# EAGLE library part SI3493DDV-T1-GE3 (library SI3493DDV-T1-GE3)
MOSFET -20V Vds 8V Vgs TSOP-6 Source: Datasheet
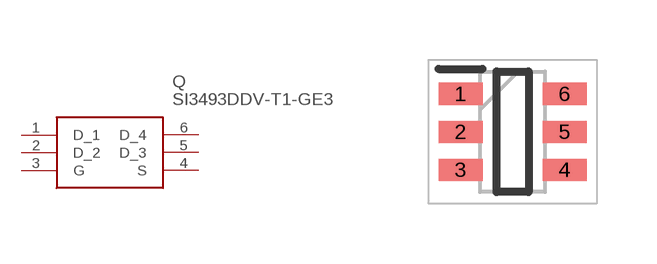
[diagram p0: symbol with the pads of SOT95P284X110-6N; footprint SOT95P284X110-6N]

Designator prefix Q

## SI3493DDV-T1-GE3 (Description: MOSFET -20V Vds 8V Vgs TSOP-6; Height: 1.1mm; Manufacturer_Name: Vishay; Manufacturer_Part_Number: SI3493DDV-T1-GE3; Mouser_Part_Number: 78-SI3493DDV-T1-GE3; Mouser_Price-Stock: https://www.mouser.co.uk/ProductDetail/Vishay-Siliconix/SI3493DDV-T1-GE3?qs=Mv7BduZupUhpV99w3U%2FyBA%3D%3D)  [SOT95P284X110-6N]
1  D_1
2  D_2
3  G
4  S
5  D_3
6  D_4

## Footprint SOT95P284X110-6N (pad centres in mm)
MO-193C
smd 1.1 x 0.55: 1 -1.3,0.95; 2 -1.3,0; 3 -1.3,-0.95; 4 1.3,-0.95; 5 1.3,0; 6 1.3,0.95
